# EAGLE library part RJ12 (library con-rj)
RJ12, RJ14 and RJ25 RJ12, RJ14 and RJ25 jacks side mounted http://www.tycoelectronics.com
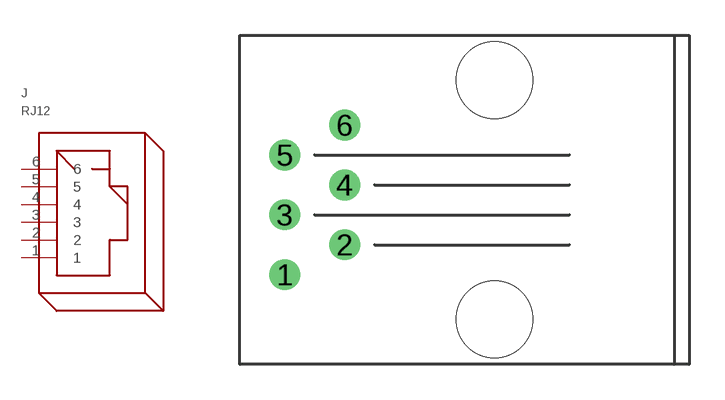
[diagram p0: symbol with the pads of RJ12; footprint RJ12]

Designator prefix J

## RJ12  [RJ12]
1  1
2  2
3  3
4  4
5  5
6  6

## Footprint RJ12 (pad centres in mm)
RJ12, RJ14, RJ25 RJ12, RJ14 and RJ22 jacks side mounted http://www.tycoelectronics.com
drill 0.8: 1 -8.89,-3.175; 2 -6.35,-1.905; 3 -8.89,-0.635; 4 -6.35,0.635; 5 -8.89,1.905; 6 -6.35,3.175
hole 3.25 at 0,-5.08
hole 3.25 at 0,5.08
